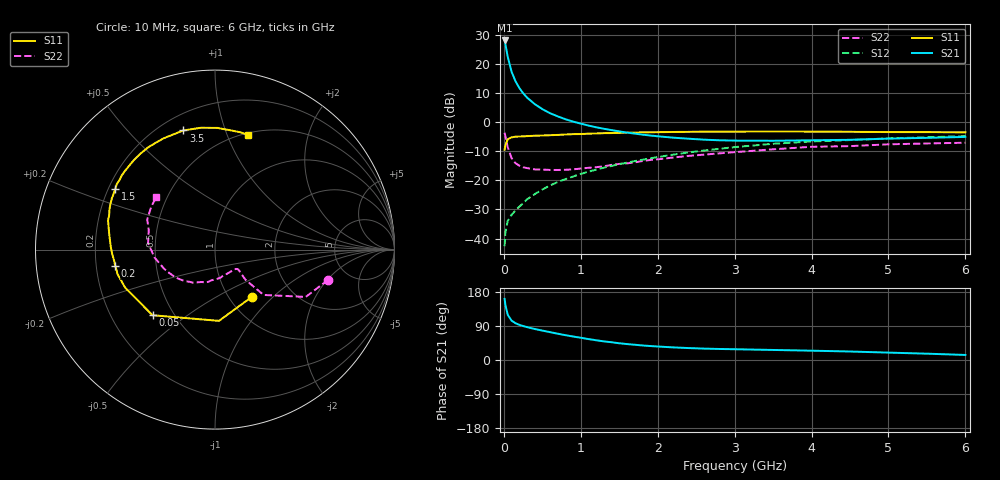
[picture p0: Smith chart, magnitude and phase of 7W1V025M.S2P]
! Infineon Technologies  Discrete & RF Semiconductors
! BFS17W
! Si NPN RF Bipolar Junction Transistor in SOT323
! VCE = 1 V  IC = 25 mA
! Common Emitter S-Parameters:  August  1999
# GHz  S  MA  R  50
!  f  S11  S21  S12  S22
! GHz  MAG  ANG  MAG  ANG  MAG  ANG  MAG  ANG
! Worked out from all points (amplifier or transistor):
!   36 points, 10 MHz to 6 GHz, reference 50 ohm
!   highest |S21| = 28.0 dB at 10 MHz (marker M1)
!   |S21| within 3 dB of that: start of sweep to 32.39 MHz
!   unconditionally stable (mu >= 1): start of sweep to 19.93 MHz; 20.21 MHz to end of sweep
!   at 250 MHz: K = 2.58, MAG = 11.9 dB, |S12| = -27.9 dB
!   at 1.4 GHz: K = 2.22, MAG = -0.1 dB, |S12| = -15.1 dB
!   at 6 GHz: K = 1.16, MAG = -2.6 dB, |S12| = -4.9 dB
!   S11 on the Smith chart (normalised r, x): 10 MHz: 1.27, -0.75; 50 MHz: 0.38, -0.37; 200 MHz: 0.28, -0.07; 1.5 GHz: 0.23, +0.26; 3.5 GHz: 0.29, +0.73; 6 GHz: 0.52, +1.19
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0.01  0.334 -51.7  25.01 161.3  0.0074 68.8  0.6522 -15.0
0.02  0.3977 -86.8  21.79 145.6  0.0126 59.9  0.5705 -27.5
0.05  0.5049 -133.6  13.18 119.5  0.02 47.0  0.3707 -43.0
0.1  0.5433 -156.9  7.312 104.0  0.0254 45.9  0.2403 -44.7
0.15  0.5596 -165.7  5.034 97.2  0.0303 49.7  0.1971 -42.6
0.2  0.5628 -170.7  3.845 92.9  0.0351 55.2  0.1785 -41.0
0.25  0.5662 -174.3  3.127 89.7  0.0404 57.7  0.167 -40.6
0.3  0.5716 -176.7  2.631 86.9  0.0468 61.0  0.1619 -41.7
0.4  0.5802 179.0  2.03 81.9  0.0576 64.1  0.1535 -45.4
0.5  0.5857 175.8  1.662 77.6  0.0694 66.0  0.1525 -49.6
0.6  0.5924 172.9  1.413 73.5  0.0815 67.0  0.1504 -54.9
0.8  0.6091 167.1  1.114 65.5  0.1046 68.1  0.1513 -67.9
1.1  0.6296 159.0  0.867 55.2  0.1404 68.0  0.1636 -85.4
1.5  0.6499 148.9  0.689 44.2  0.1886 66.0  0.1907 -106.7
1.8  0.664 141.6  0.607 38.4  0.2247 63.7  0.2132 -120.3
2.2  0.6731 132.1  0.538 33.3  0.2749 60.0  0.2453 -134.8
2.8  0.6807 118.7  0.485 29.1  0.3463 53.2  0.289 -154.1
3.5  0.6868 104.9  0.476 26.5  0.4224 44.3  0.3397 -172.5
4  0.6834 96.7  0.485 24.6  0.4627 37.6  0.3748 174.4
4.5  0.6784 89.1  0.494 22.4  0.489 31.9  0.3851 163.4
5.5  0.6691 78.0  0.534 16.7  0.5456 22.2  0.4279 146.2
6  0.6644 73.7  0.554 13.3  0.5712 17.5  0.4401 137.9
